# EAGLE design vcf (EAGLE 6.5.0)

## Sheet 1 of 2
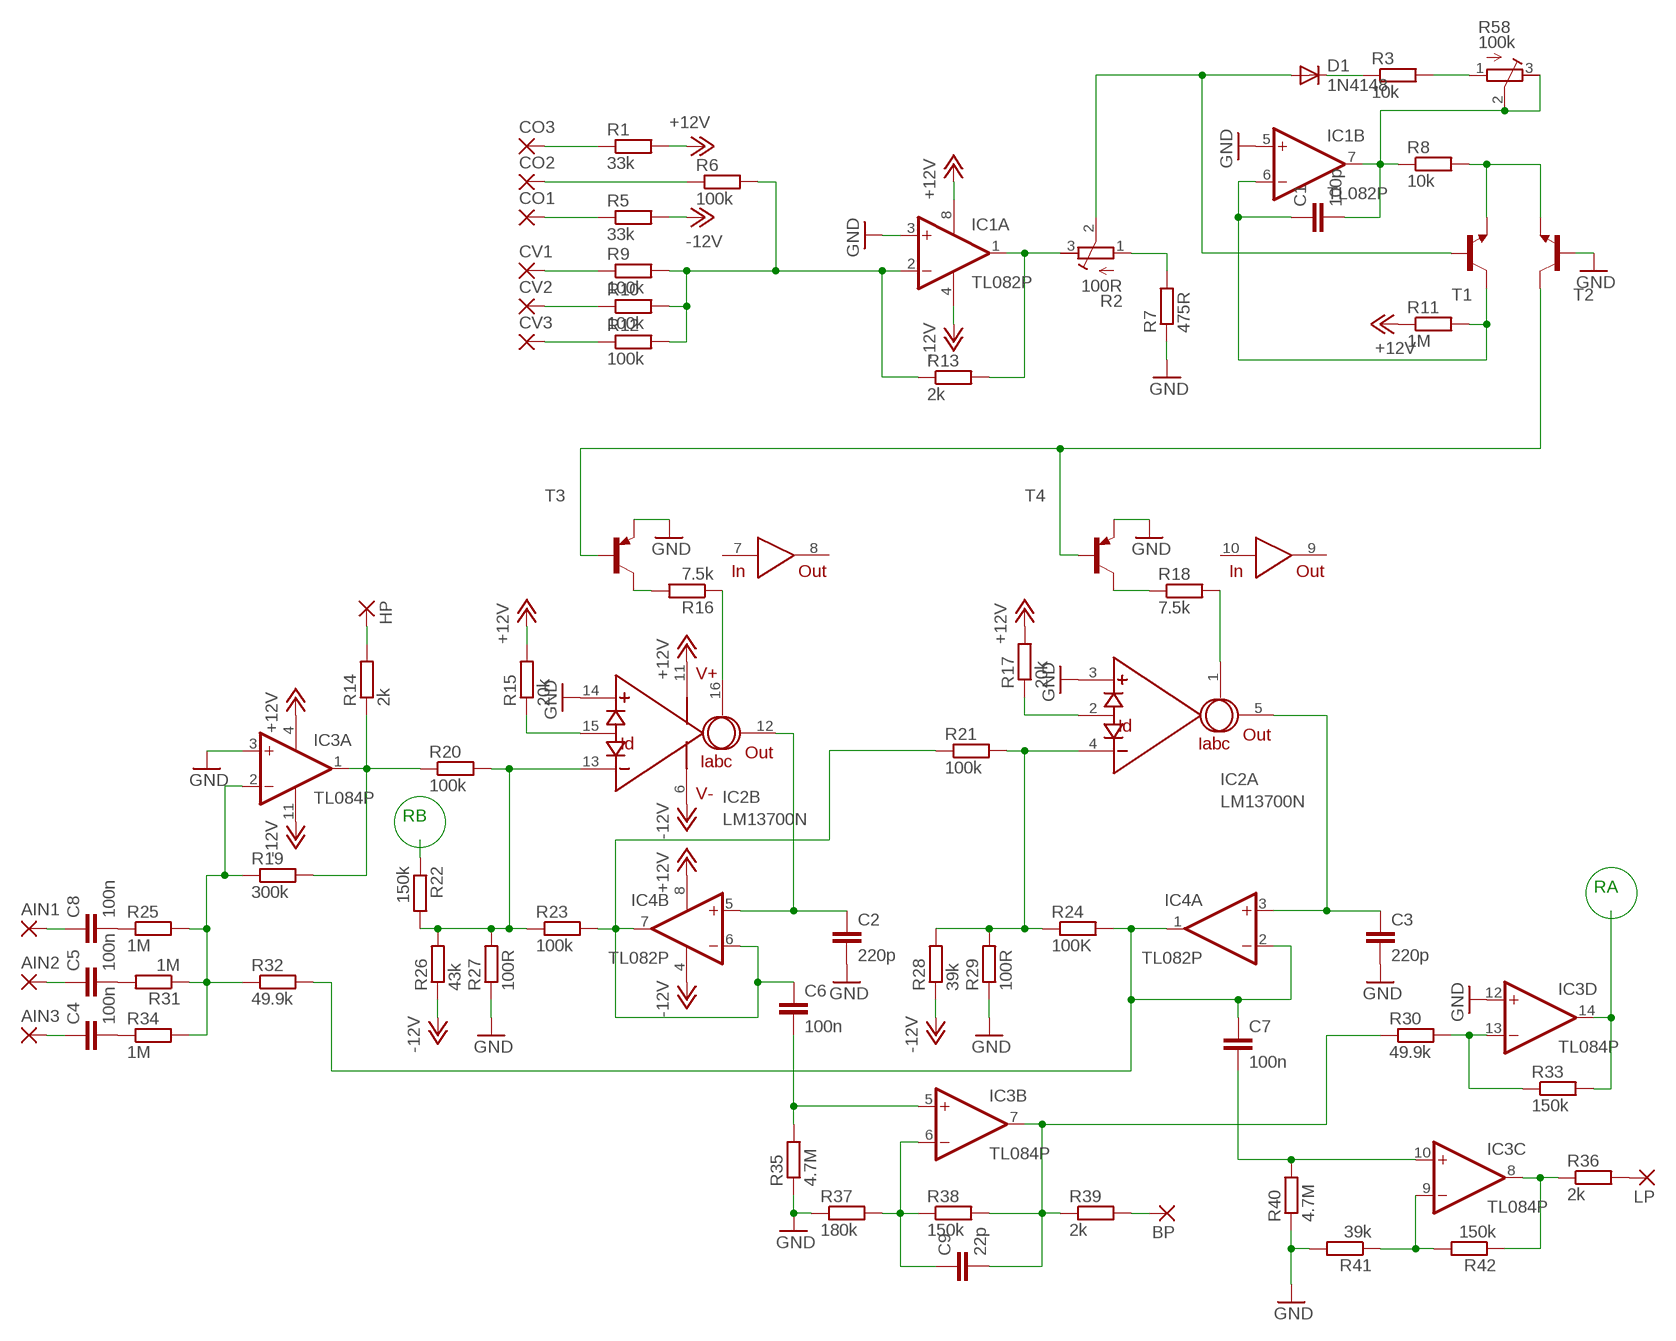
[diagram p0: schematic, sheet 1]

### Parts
AIN1  2,54/1,0  [2,54/1,0]
AIN2  2,54/1,0  [2,54/1,0]
AIN3  2,54/1,0  [2,54/1,0]
BP  2,54/1,0  [2,54/1,0]
C1  100p  C-EU050-035X075  [C050-035X075]
C2  220p  C-EU050-035X075  [C050-035X075]
C3  220p  C-EU050-035X075  [C050-035X075]
C4  100n  C-EU050-035X075  [C050-035X075]
C5  100n  C-EU050-035X075  [C050-035X075]
C6  100n  C-EU050-035X075  [C050-035X075]
C7  100n  C-EU050-035X075  [C050-035X075]
C8  100n  C-EU050-035X075  [C050-035X075]
C9  22p  C-EU050-035X075  [C050-035X075]
CO1  2,54/1,0  [2,54/1,0]
CO2  2,54/1,0  [2,54/1,0]
CO3  2,54/1,0  [2,54/1,0]
CV1  2,54/1,0  [2,54/1,0]
CV2  2,54/1,0  [2,54/1,0]
CV3  2,54/1,0  [2,54/1,0]
D1  1N4148  1N4148DO35-7  [DO35-7]
HP  2,54/1,0  [2,54/1,0]
IC1  TL082P  [DIL08]
IC2  LM13700N  [DIL16]
IC3  TL084P  [DIL14]
IC4  TL082P  [DIL08]
LP  2,54/1,0  [2,54/1,0]
R1  33k  R-EU_0309/10  [0309/10]
R2  100R  R-TRIMM64W  [RTRIM64W]
R3  10k  R-EU_0309/10  [0309/10]
R5  33k  R-EU_0309/10  [0309/10]
R6  100k  R-EU_0309/10  [0309/10]
R7  475R  R-EU_0309/10  [0309/10]
R8  10k  R-EU_0309/10  [0309/10]
R9  100k  R-EU_0309/10  [0309/10]
R10  100k  R-EU_0309/10  [0309/10]
R11  1M  R-EU_0309/10  [0309/10]
R12  100k  R-EU_0309/10  [0309/10]
R13  2k  R-EU_0309/10  [0309/10]
R14  2k  R-EU_0309/10  [0309/10]
R15  20k  R-EU_0309/10  [0309/10]
R16  7.5k  R-EU_0309/10  [0309/10]
R17  20k  R-EU_0309/10  [0309/10]
R18  7.5k  R-EU_0309/10  [0309/10]
R19  300k  R-EU_0309/10  [0309/10]
R20  100k  R-EU_0309/10  [0309/10]
R21  100k  R-EU_0309/10  [0309/10]
R22  150k  R-EU_0309/10  [0309/10]
R23  100k  R-EU_0309/10  [0309/10]
R24  100K  R-EU_0309/10  [0309/10]
R25  1M  R-EU_0309/10  [0309/10]
R26  43k  R-EU_0309/10  [0309/10]
R27  100R  R-EU_0309/10  [0309/10]
R28  39k  R-EU_0309/10  [0309/10]
R29  100R  R-EU_0309/10  [0309/10]
R30  49.9k  R-EU_0309/10  [0309/10]
R31  1M  R-EU_0309/10  [0309/10]
R32  49.9k  R-EU_0309/10  [0309/10]
R33  150k  R-EU_0309/10  [0309/10]
R34  1M  R-EU_0309/10  [0309/10]
R35  4.7M  R-EU_0309/10  [0309/10]
R36  2k  R-EU_0309/10  [0309/10]
R37  180k  R-EU_0309/10  [0309/10]
R38  150k  R-EU_0309/10  [0309/10]
R39  2k  R-EU_0309/10  [0309/10]
R40  4.7M  R-EU_0309/10  [0309/10]
R41  39k  R-EU_0309/10  [0309/10]
R42  150k  R-EU_0309/10  [0309/10]
R58  100k  R-TRIMM64W  [RTRIM64W]
T1  2N3904-NPN-TO92-EBC  [TO92-EBC]
T2  2N3904-NPN-TO92-EBC  [TO92-EBC]
T3  2N3906-PNP-TO92-EBC  [TO92-EBC]
T4  2N3906-PNP-TO92-EBC  [TO92-EBC]

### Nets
+12V: IC1.8(P:V+) IC2.11(V+) IC3.4(P:V+) IC4.8(P:V+) R1.2 R11.1 R15.2 R17.2 ; also sheet 2
-12V: IC1.4(P:V-) IC2.6(V-) IC3.11(P:V-) IC4.4(P:V-) R5.2 R26.1 R28.1 ; also sheet 2
GND: C2.2 C3.2 IC1.3(A:+IN) IC1.5(B:+IN) IC2.3(A:+IN) IC2.14(B:+IN) IC3.3(A:+IN) IC3.12(D:+IN) R7.1 R27.1 R29.1 R35.1 R37.1 R40.1 R41.2 T2.B T3.E T4.E ; also sheet 2
N$13: CO3.1(P) R1.1
N$14: CO2.1(P) R6.1
N$15: CO1.1(P) R5.1
N$16: CV1.1(P) R9.1
N$17: CV2.1(P) R10.1
N$18: CV3.1(P) R12.1
N$19: IC1.2(A:-IN) R6.2 R9.2 R10.2 R12.2 R13.1
N$20: IC1.1(A:OUT) R2.3(E) R13.2
N$21: R2.1(A) R7.2
N$22: C8.2 R25.1
N$23: R8.2 T1.E T2.E
N$24: C1.1 IC1.6(B:-IN) R11.2 T1.C
N$25: D1.C R3.1
N$26: R3.2 R58.1(A)
N$27: C1.2 IC1.7(B:OUT) R8.1 R58.2(S) R58.3(E)
N$28: D1.A R2.2(S) T1.B
N$29: T2.C T3.B T4.B
N$30: C6.2 IC3.5(B:+IN) R35.2
N$31: C5.2 R31.2
N$32: C4.2 R34.1
N$33: IC3.1(A:OUT) R14.1 R19.2 R20.1
N$34: HP.1(P) R14.2
N$35: IC3.2(A:-IN) R19.1 R25.2 R31.1 R32.1 R34.2
N$36: IC2.13(B:-IN) R20.2 R22.2 R23.1 R26.2 R27.2
N$37: IC2.15(B:ID) R15.1
N$38: IC2.2(A:ID) R17.1
N$39: IC2.16(B:IABC) R16.1
N$40: R16.2 T3.C
N$41: R18.1 T4.C
N$42: IC2.1(A:IABC) R18.2
N$43: IC2.4(A:-IN) R21.2 R24.1 R28.2 R29.2
N$44: C6.1 IC4.6(B:-IN) IC4.7(B:OUT) R21.1 R23.2
N$45: C2.1 IC2.12(B:OUT) IC4.5(B:+IN)
N$46: C3.1 IC2.5(A:OUT) IC4.3(A:+IN)
N$47: AIN1.1(P) C8.1
N$48: C9.1 IC3.6(B:-IN) R37.2 R38.1
N$50: C9.2 IC3.7(B:OUT) R30.1 R38.2 R39.1
N$51: BP.1(P) R39.2
N$52: IC3.13(D:-IN) R30.2 R33.1
N$53: AIN2.1(P) C5.1
N$54: C7.2 IC3.10(C:+IN) R40.2
N$55: IC3.9(C:-IN) R41.1 R42.2
N$56: IC3.8(C:OUT) R36.1 R42.1
N$57: LP.1(P) R36.2
N$58: AIN3.1(P) C4.1
N$59: C7.1 IC4.1(A:OUT) IC4.2(A:-IN) R24.2 R32.2
RA: IC3.14(D:OUT) R33.2 ; also sheet 2
RB: R22.1 ; also sheet 2
Unconnected: IC2.7(IN) IC2.8(OUT) IC2.9(OUT) IC2.10(IN)

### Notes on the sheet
- RB
- RA

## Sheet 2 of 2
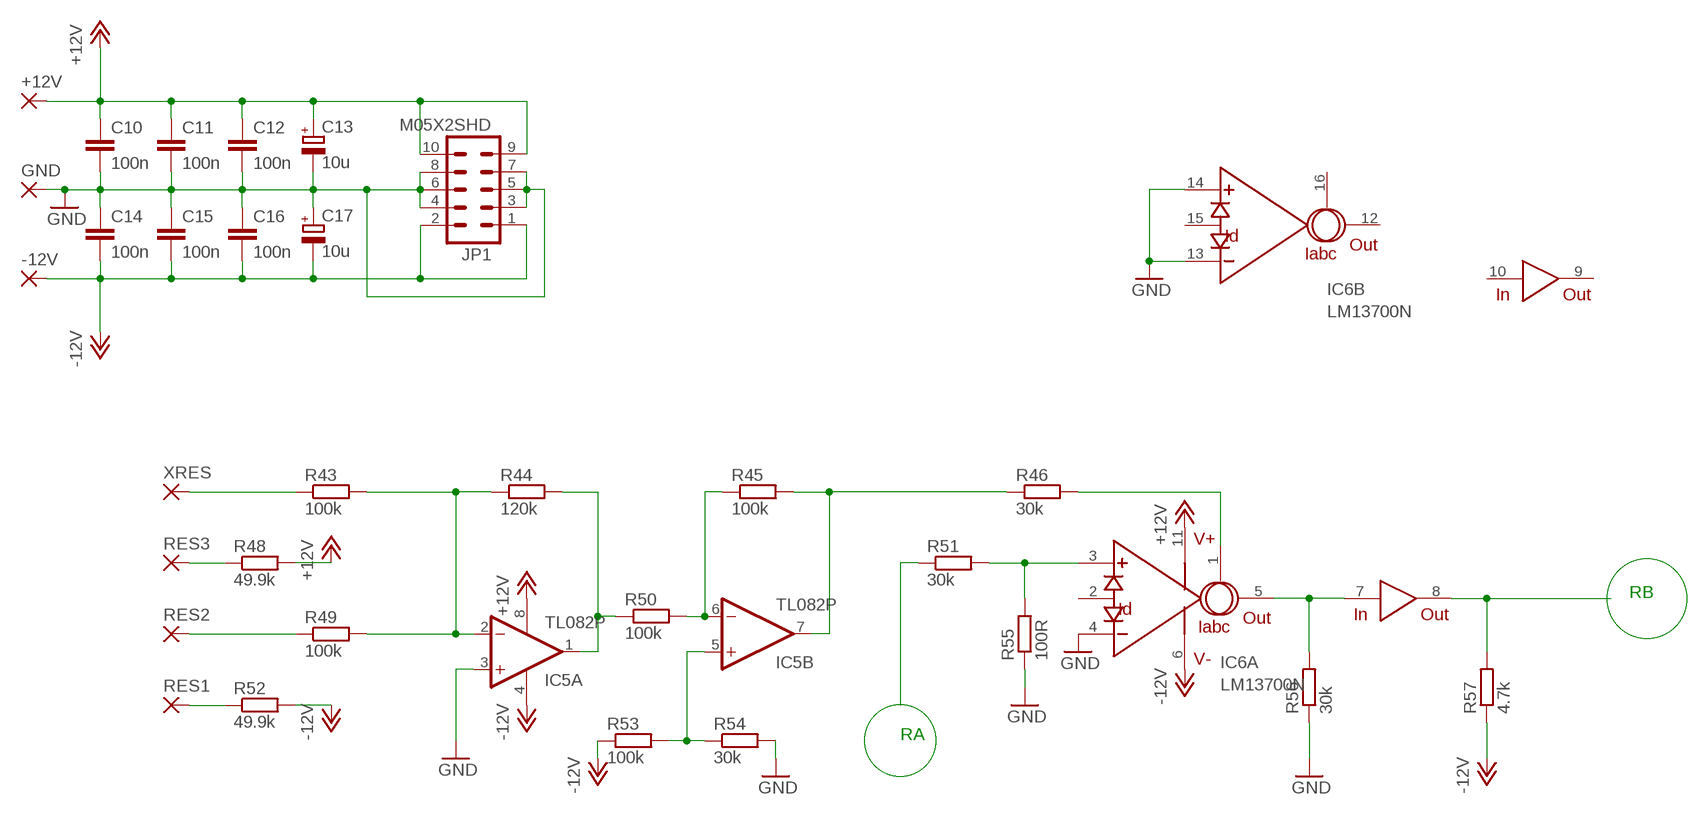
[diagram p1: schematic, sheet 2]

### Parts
+12V  2,54/1,0  [2,54/1,0]
-12V  2,54/1,0  [2,54/1,0]
C10  100n  C-EU050-035X075  [C050-035X075]
C11  100n  C-EU050-035X075  [C050-035X075]
C12  100n  C-EU050-035X075  [C050-035X075]
C13  10u  CPOL-EUE3.5-8  [E3,5-8]
C14  100n  C-EU050-035X075  [C050-035X075]
C15  100n  C-EU050-035X075  [C050-035X075]
C16  100n  C-EU050-035X075  [C050-035X075]
C17  10u  CPOL-EUE3.5-8  [E3,5-8]
GND  2,54/1,0  [2,54/1,0]
IC5  TL082P  [DIL08]
IC6  LM13700N  [DIL16]
JP1  M05X2SHD  [2X5-SHROUDED]
R43  100k  R-EU_0309/10  [0309/10]
R44  120k  R-EU_0309/10  [0309/10]
R45  100k  R-EU_0309/10  [0309/10]
R46  30k  R-EU_0309/10  [0309/10]
R48  49.9k  R-EU_0309/10  [0309/10]
R49  100k  R-EU_0309/10  [0309/10]
R50  100k  R-EU_0309/10  [0309/10]
R51  30k  R-EU_0309/10  [0309/10]
R52  49.9k  R-EU_0309/10  [0309/10]
R53  100k  R-EU_0309/10  [0309/10]
R54  30k  R-EU_0309/10  [0309/10]
R55  100R  R-EU_0309/10  [0309/10]
R56  30k  R-EU_0309/10  [0309/10]
R57  4.7k  R-EU_0309/10  [0309/10]
RES1  2,54/1,0  [2,54/1,0]
RES2  2,54/1,0  [2,54/1,0]
RES3  2,54/1,0  [2,54/1,0]
XRES  2,54/1,0  [2,54/1,0]

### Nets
+12V: +12V.1(P) C10.1 C11.1 C12.1 C13.+ IC5.8(P:V+) IC6.11(V+) JP1.9 JP1.10 R48.2 ; also sheet 1
-12V: -12V.1(P) C14.2 C15.2 C16.2 C17.- IC5.4(P:V-) IC6.6(V-) JP1.1 JP1.2 R52.2 R53.1 R57.1 ; also sheet 1
GND: C10.2 C11.2 C12.2 C13.- C14.1 C15.1 C16.1 C17.+ GND.1(P) IC5.3(A:+IN) IC6.4(A:-IN) IC6.13(B:-IN) IC6.14(B:+IN) JP1.3 JP1.4 JP1.5 JP1.6 JP1.7 JP1.8 R54.2 R55.1 R56.1 ; also sheet 1
N$1: R43.1 XRES.1(P)
N$2: R48.1 RES3.1(P)
N$3: R52.1 RES1.1(P)
N$4: R49.1 RES2.1(P)
N$5: IC5.2(A:-IN) R43.2 R44.1 R49.2
N$6: IC5.1(A:OUT) R44.2 R50.1
N$7: IC5.6(B:-IN) R45.1 R50.2
N$8: IC5.5(B:+IN) R53.2 R54.1
N$9: IC6.1(A:IABC) R46.2
N$10: IC5.7(B:OUT) R45.2 R46.1
N$11: IC6.3(A:+IN) R51.2 R55.2
N$12: IC6.5(A:OUT) IC6.7(IN) R56.2
RA: R51.1 ; also sheet 1
RB: IC6.8(OUT) R57.2 ; also sheet 1
Unconnected: IC6.2(A:ID) IC6.9(OUT) IC6.10(IN) IC6.12(B:OUT) IC6.15(B:ID) IC6.16(B:IABC)

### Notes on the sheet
- RB
- RA

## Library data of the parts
+12V -12V AIN1-AIN3 BP CO1-CO3 CV1-CV3 GND HP LP RES1-RES3 XRES = wirepad:2,54/1,0: THROUGH-HOLE PAD
C1-C12 C14-C16 = rcl:C-EU: CAPACITOR, European symbol
C13 C17 = rcl:CPOL-EU: POLARIZED CAPACITOR, European symbol
D1 = diode:1N4148: DIODE
IC1 IC4 IC5 = cavalier:TL082: OP AMP
IC2 IC6 = synthdiy:LM13700: National Dual OTA with buffers.
IC3 = cavalier:TL084: OP AMP
JP1 = SparkFun:M05X2: Header 5x2 Standard 10-pin dual row 0.1" header. Commonly used with AVR-ISP. Use with Spark Fun Electronics SKU: PRT-00778
R1 R3 R5-R46 R48-R57 = rcl:R-EU_: RESISTOR, European symbol
R2 R58 = rcl:R-TRIMM: Trimm resistor
T1 T2 = transistor-neu-to92:*-NPN-: NPN Transistror
T3 T4 = transistor-neu-to92:*-PNP-: PNP Transistror

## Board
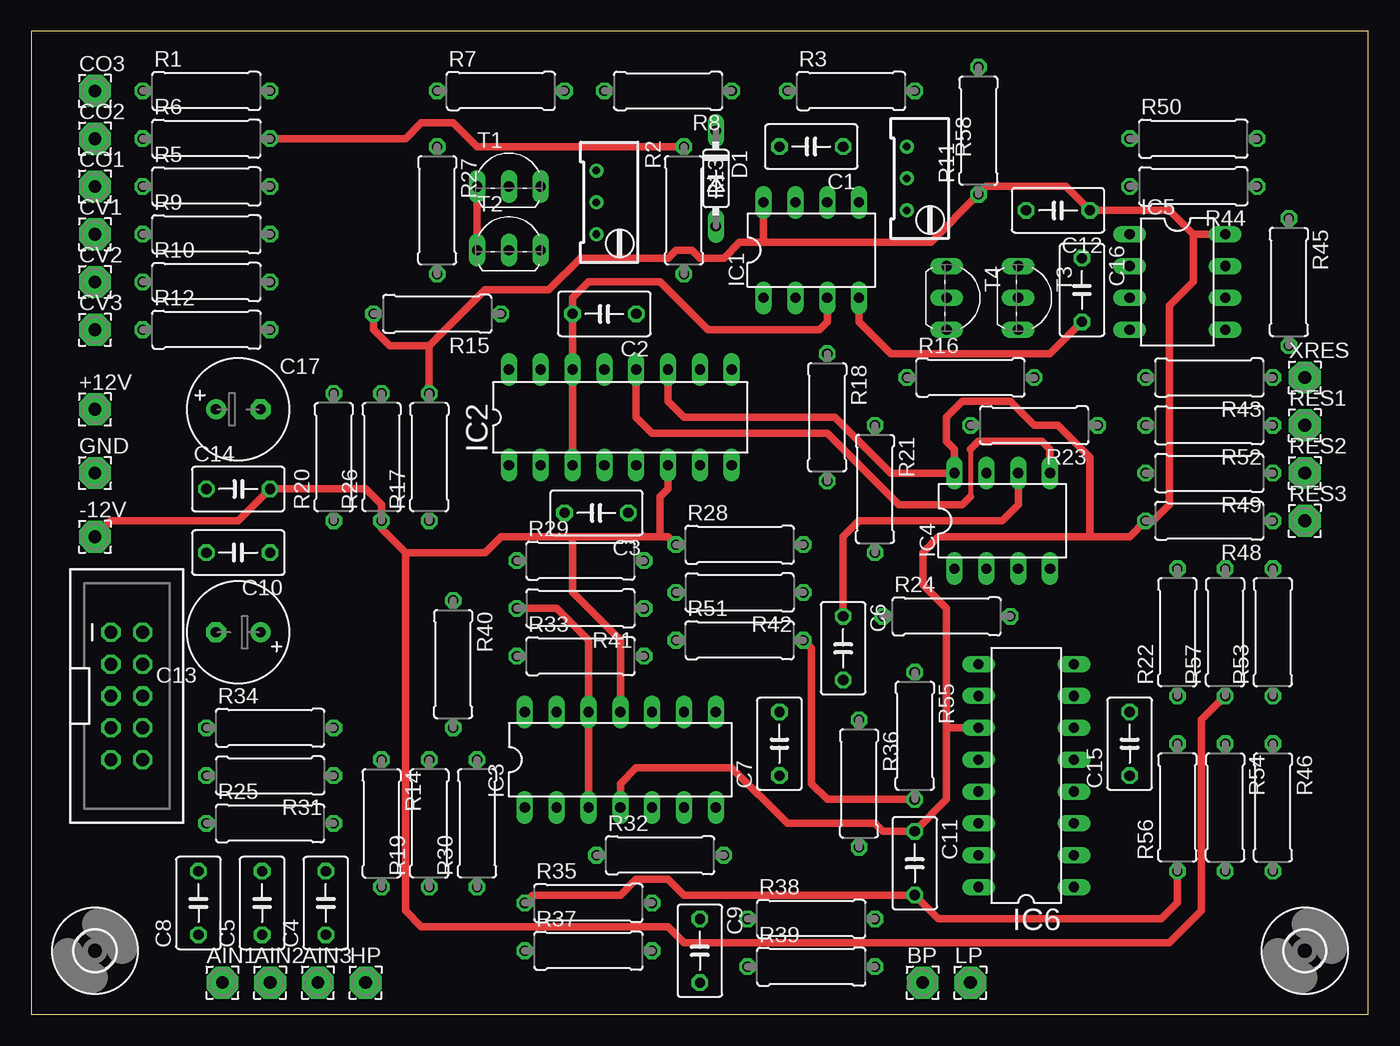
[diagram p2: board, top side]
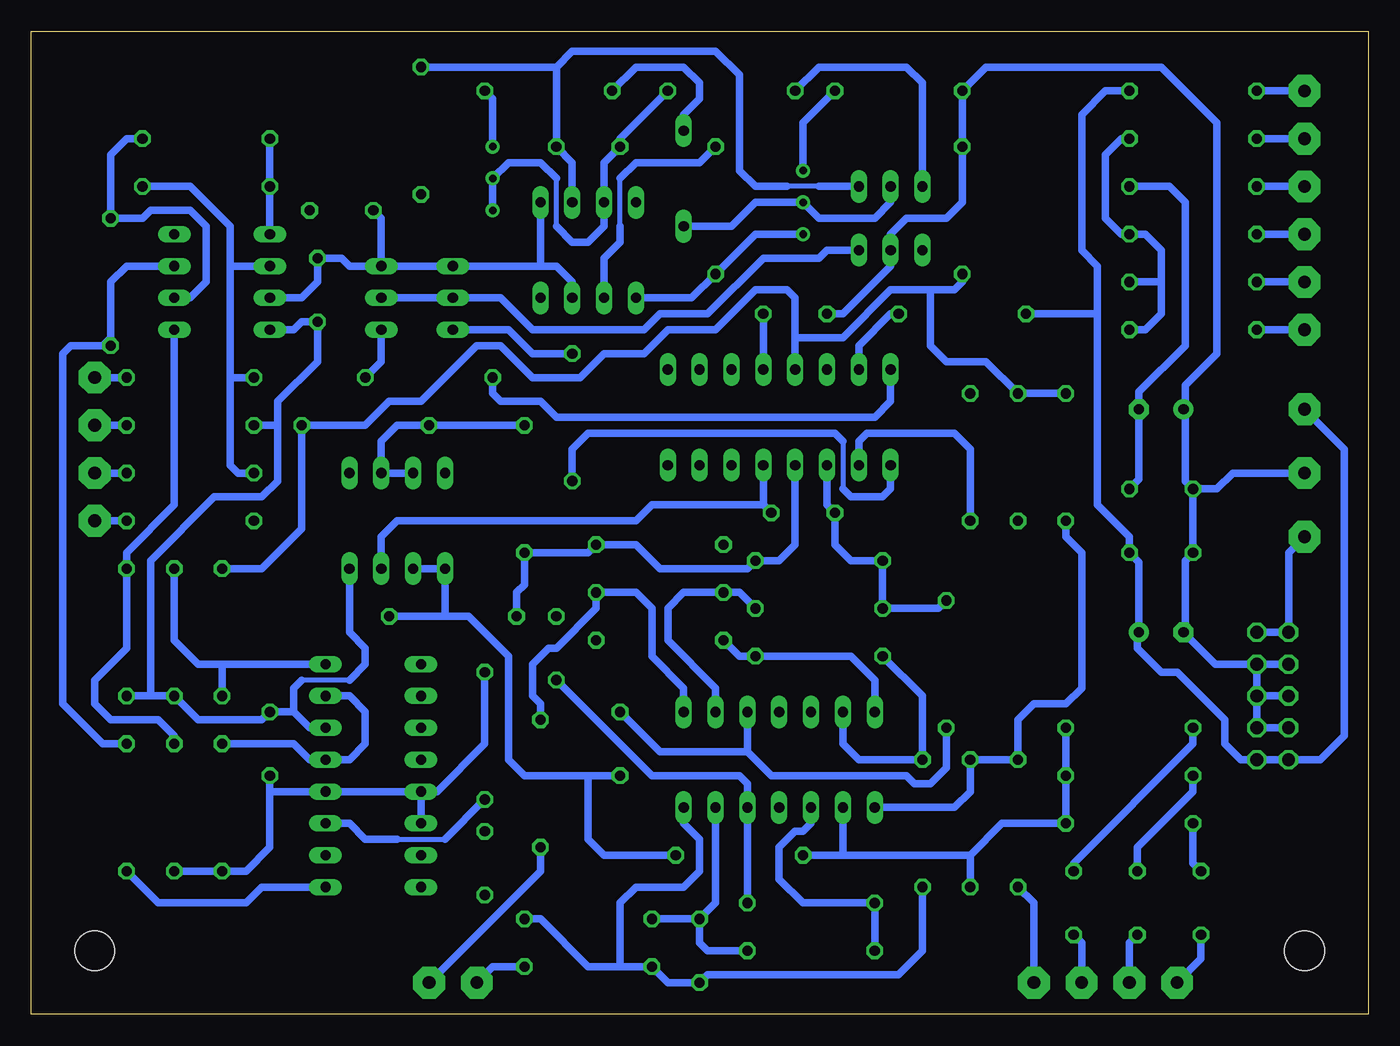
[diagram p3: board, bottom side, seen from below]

Size 106.66 x 78.41 mm. Coordinates in mm from the lower left corner, seen from the top.
Outline: 0,0 106.66,0 106.66,78.41 0,78.41 0,0
Copper layers (1*16): Top 0.035mm / dielectric 1.5mm / Bottom 0.035mm
Design rules "default": minimum track width 10mil, minimum drill 24mil, track to track 8mil, track to pad 8mil, pad to pad 8mil, via to via 8mil, smd to smd 8mil, copper to edge 40mil, drill to drill 8mil, minimum pad ring 10mil, minimum via ring 8mil, stop-mask expansion 4mil, vias tented up to drill 0mil, thermal gap 10mil

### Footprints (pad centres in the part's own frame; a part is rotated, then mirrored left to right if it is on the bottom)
2,54/1,0 = drill 1.016 pad 2.54 octagon: 1 0,0
C050-035X075 = drill 0.813 octagon: 1 -2.54,0; 2 2.54,0
E3,5-8 = drill 0.813 pad 1.6: + -1.778,0 | drill 0.813 pad 1.6 octagon: - 1.778,0
DO35-7 = drill 0.813 long: A 3.81,0; C -3.81,0
DIL08 = drill 0.813 pad 1.27 long: 1 -3.81,-3.81; 2 -1.27,-3.81; 3 1.27,-3.81; 4 3.81,-3.81; 5 3.81,3.81; 6 1.27,3.81; 7 -1.27,3.81; 8 -3.81,3.81
DIL16 = drill 0.813 long: 1 -8.89,-3.81; 2 -6.35,-3.81; 3 -3.81,-3.81; 4 -1.27,-3.81; 5 1.27,-3.81; 6 3.81,-3.81; 7 6.35,-3.81; 8 8.89,-3.81; 9 8.89,3.81; 10 6.35,3.81; 11 3.81,3.81; 12 1.27,3.81; 13 -1.27,3.81; 14 -3.81,3.81; 15 -6.35,3.81; 16 -8.89,3.81
DIL14 = drill 0.813 long: 1 -7.62,-3.81; 2 -5.08,-3.81; 3 -2.54,-3.81; 4 0,-3.81; 5 2.54,-3.81; 6 5.08,-3.81; 7 7.62,-3.81; 8 7.62,3.81; 9 5.08,3.81; 10 2.54,3.81; 11 0,3.81; 12 -2.54,3.81; 13 -5.08,3.81; 14 -7.62,3.81
2X5-SHROUDED = drill 1.016 octagon: 1 -1.27,5.08; 2 1.27,5.08; 3 -1.27,2.54; 4 1.27,2.54; 5 -1.27,0; 6 1.27,0; 7 -1.27,-2.54; 8 1.27,-2.54; 9 -1.27,-5.08; 10 1.27,-5.08
0309/10 = drill 0.813 octagon: 1 -5.08,0; 2 5.08,0
RTRIM64W = drill 0.61: 1 1.27,-2.54; 2 1.27,0; 3 1.27,2.54
TO92-EBC = drill 0.813 long: B 0,-1.27; C 2.54,-1.27; E -2.54,-1.27
3,2 = hole 3.2: 0,0

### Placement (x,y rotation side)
+12V  5.08,48.26 0 top
-12V  5.08,38.1 0 top
AIN1  15.24,2.54 0 top
AIN2  19.05,2.54 0 top
AIN3  22.86,2.54 0 top
BP  71.12,2.54 0 top
C1  62.23,69.22 180 top
C2  45.72,55.88 180 top
C3  45.09,40.01 180 top
C4  23.5,8.89 90 top
C5  18.41,8.89 90 top
C6  64.77,29.21 270 top
C7  59.69,21.59 90 top
C8  13.34,8.89 90 top
C9  53.34,5.08 270 top
C10  16.51,36.83 180 top
C11  70.48,12.06 270 top
C12  81.92,64.14 180 top
C13  16.51,30.48 180 top
C14  16.51,41.91 0 top
C15  87.63,21.59 90 top
C16  83.82,57.78 270 top
C17  16.51,48.26 0 top
CO1  5.08,66.04 0 top
CO2  5.08,69.85 0 top
CO3  5.08,73.66 0 top
CV1  5.08,62.23 0 top
CV2  5.08,58.42 0 top
CV3  5.08,54.61 0 top
D1  54.61,66.67 270 top
GND  5.08,43.18 0 top
HP  26.67,2.54 0 top
IC1  62.23,60.96 0 top
IC2  46.99,47.62 0 top
IC3  46.99,20.32 0 top
IC4  77.47,39.37 0 top
IC5  91.44,58.42 270 top
IC6  79.38,19.05 90 top
JP1  7.62,25.4 0 top
LP  74.93,2.54 0 top
R1  13.97,73.66 0 top
R2  46.35,64.77 180 top
R3  65.41,73.66 0 top
R5  13.97,66.04 0 top
R6  13.97,69.85 0 top
R7  37.47,73.66 0 top
R8  50.8,73.66 180 top
R9  13.97,62.23 0 top
R10  13.97,58.42 0 top
R11  75.56,70.48 90 top
R12  13.97,54.61 0 top
R13  52.07,64.14 270 top
R14  27.94,15.24 270 top
R15  32.38,55.88 180 top
R16  74.93,50.8 0 top
R17  31.75,44.45 90 top
R18  63.5,47.62 270 top
R19  31.75,15.24 90 top
R20  24.13,44.45 90 top
R21  67.31,41.91 270 top
R22  91.44,30.48 90 top
R23  80.01,46.99 180 top
R24  73.03,31.75 0 top
R25  19.05,15.24 0 top
R26  27.94,44.45 90 top
R27  32.38,64.14 270 top
R28  56.52,37.47 0 top
R29  43.81,36.2 0 top
R30  35.56,15.24 90 top
R31  19.05,19.05 180 top
R32  50.16,12.7 0 top
R33  43.81,28.57 0 top
R34  19.05,22.86 0 top
R35  44.45,8.89 0 top
R36  66.04,18.41 270 top
R37  44.45,5.08 0 top
R38  62.23,7.62 0 top
R39  62.23,3.81 0 top
R40  33.66,27.94 270 top
R41  43.81,32.38 180 top
R42  56.52,33.66 180 top
R43  93.98,50.8 180 top
R44  92.71,66.04 180 top
R45  100.33,58.42 270 top
R46  99.06,16.51 270 top
R48  93.98,39.37 180 top
R49  93.98,43.18 180 top
R50  92.71,69.85 0 top
R51  56.52,29.84 0 top
R52  93.98,46.99 180 top
R53  99.06,30.48 90 top
R54  95.25,16.51 270 top
R55  70.48,22.23 270 top
R56  91.44,16.51 90 top
R57  95.25,30.48 90 top
R58  71.12,66.67 180 top
RES1  101.6,46.99 0 top
RES2  101.6,43.18 0 top
RES3  101.6,39.37 0 top
T1  38.1,67.31 0 top
T2  38.1,62.23 0 top
T3  80.01,57.15 270 top
T4  74.3,57.15 270 top
U$1  [3,2]  5.08,5.08 0 top
U$2  [3,2]  101.6,5.08 0 top
XRES  101.6,50.8 0 top

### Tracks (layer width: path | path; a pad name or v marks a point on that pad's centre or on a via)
+12V
  Top 0.61: IC3.4 46.99,18.41 48.26,19.68 55.88,19.68 60.33,15.24 67.31,15.24 67.94,14.61 C11.1 73.03,17.14 73.03,22.86 | 73.03,22.86 73.03,32.38 71.12,34.29 71.12,36.83 72.39,38.1 84.45,38.1 | R15.2 27.3,54.61 28.57,53.34 31.75,53.34 | 92.71,62.23 90.81,64.14 C12.1 82.55,66.04 76.2,66.04 R11.1 71.75,61.59 58.42,61.59 | 92.71,62.23 IC5.8 | IC6.11 73.03,22.86 | 92.71,62.23 92.71,58.42 90.81,56.52 90.81,40.64 89.53,39.37 R48.2 87.63,38.1 84.45,38.1 | IC1.8 58.42,61.59 | IC2.11 50.8,48.9 52.07,47.62 64.14,47.62 68.58,43.18 IC4.8 73.66,45.09 73.03,45.72 73.03,47.62 74.3,48.9 78.11,48.9 80.01,46.99 81.92,46.99 84.45,44.45 84.45,38.1 | R17.2 31.75,53.34 | 58.42,61.59 56.52,61.59 55.24,60.33 53.34,60.33 52.7,60.96 51.44,60.96 50.8,60.33 43.81,60.33 41.27,57.78 36.2,57.78 31.75,53.34
  Bottom 0.61: +12V.1 1.91,45.09 1.91,22.23 3.81,20.32 JP1.9 JP1.10 10.16,20.32 11.43,21.59 11.43,23.5 15.24,27.3 16.51,27.3 18.41,29.21 18.41,30.35 C13.+ 18.29,36.07 C10.1 19.05,38.1 21.59,40.64 21.59,55.88 | 21.59,55.88 21.59,59.69 22.86,60.96 22.86,71.75 20.95,73.66 R1.2 | 21.59,55.88 R15.2
-12V
  Top 0.61: 29.84,36.83 36.2,36.83 37.47,38.1 43.18,38.1 | 43.18,38.1 50.16,38.1 | IC2.6 50.8,41.91 50.16,41.27 50.16,38.1 | IC3.11 46.99,29.84 43.18,33.66 43.18,38.1 | IC1.4 66.04,55.24 68.58,52.7 81.28,52.7 C16.2 | R57.1 93.34,23.5 93.34,8.26 90.81,5.71 52.07,5.71 50.8,6.99 31.11,6.99 29.84,8.26 29.84,36.83 | 50.16,38.1 50.8,38.1 R28.1 | 29.84,36.83 27.94,38.73 R26.1 27.94,40.64 26.67,41.91 C14.2 16.51,39.37 6.35,39.37 -12V.1
  Bottom 0.406: 81.28,26.67 85.09,26.67
  Bottom 0.61: JP1.2 JP1.1 6.35,36.83 -12V.1 | R53.1 97.16,25.4 | 97.16,25.4 R57.1 93.34,23.5 88.27,23.5 C15.2 85.72,24.13 | C14.2 18.29,42.67 C17.- 18.29,49.66 14.61,53.34 14.61,64.77 15.88,66.04 R5.2 | IC6.6 84.45,22.86 85.72,24.13 | R52.2 87,46.99 | 87,46.99 87,42.55 88.27,41.27 92.08,41.27 97.16,36.2 97.16,25.4 | IC4.4 81.28,30.48 80.01,29.21 80.01,27.94 81.28,26.67 | 85.09,26.67 85.72,26.04 85.72,24.13 | 87,46.99 87,48.9 83.82,52.07 C16.2 85.09,55.24 85.72,54.61 IC5.4
GND
  Top 0.61: IC3.3 IC3.12 44.45,29.84 41.91,32.38 R41.2 | R56.1 91.44,8.89 90.17,7.62 72.39,7.62 C11.2 52.07,9.53 50.8,10.79 48.26,10.79 46.99,9.53 40.01,9.53 R35.1 | IC2.3 IC2.14 C2.2 43.18,57.15 44.45,58.42 50.16,58.42 53.98,54.61 62.87,54.61 63.5,55.24 IC1.3
  Bottom 0.61: JP1.7 JP1.8 JP1.6 | JP1.5 JP1.6 | JP1.3 JP1.4 | JP1.6 JP1.4 | R37.1 R35.1 45.09,8.89 46.99,10.79 46.99,13.34 45.72,14.61 45.09,14.61 44.45,15.24 IC3.3 | R54.2 R56.1 89.53,11.43 87.63,13.34 87.63,17.78 | IC6.13 IC6.4 87.63,17.78 | IC6.13 IC6.14 | IC6.13 74.3,17.78 70.48,21.59 R55.1 | T3.E T4.E 66.04,59.69 | 66.04,59.69 64.77,59.69 63.5,58.42 IC1.3 | IC1.5 66.04,59.69 | GND.1 10.79,43.18 12.06,41.91 C14.1 | C14.1 C10.2 14.61,36.2 14.61,30.61 C13.- 12.19,27.94 JP1.4 | C14.1 14.61,42.55 14.61,48.13 C17.+ 14.61,48.26 14.61,50.16 12.06,52.7 12.06,71.12 16.51,75.56 30.48,75.56 R7.1 R27.1 32.38,64.77 33.66,63.5 36.83,63.5 38.1,62.23 T2.B 38.1,59.69 41.91,55.88 C2.2 | R40.1 34.29,32.38 R41.2 R29.1 41.27,36.2 42.55,37.47 C3.2 43.18,40.64 IC2.3 | C12.2 78.74,63.5 T3.E | IC5.3 85.09,57.15 83.82,58.42 C16.1 81.92,60.33 81.28,59.69 T3.E | 87.63,17.78 C15.1
N$1
  Bottom 0.61: XRES.1 R43.1
N$2
  Bottom 0.61: RES3.1 R48.1
N$3
  Bottom 0.61: RES1.1 R52.1
N$4
  Bottom 0.61: RES2.1 R49.1
N$5
  Bottom 0.61: R44.1 93.98,66.04 90.81,62.87 90.81,59.69 | IC5.2 90.81,59.69 | 90.81,59.69 90.81,50.8 | 90.81,50.8 R43.2 | R49.2 90.17,43.18 90.81,43.81 90.81,50.8
N$6
  Bottom 0.61: IC5.1 R44.2 R50.1
N$7
  Bottom 0.61: IC5.6 93.98,57.15 92.71,58.42 92.71,62.87 93.98,64.14 97.16,64.14 97.79,63.5 R45.1 100.33,68.58 99.06,69.85 R50.2
N$8
  Bottom 0.61: R54.1 95.25,22.23 96.52,23.5 100.33,23.5 101.6,24.77 101.6,26.67 99.06,29.21 R53.2 99.06,36.83 95.25,40.64 IC5.5
N$9
  Bottom 0.61: IC6.1 88.27,10.16 89.53,8.89 96.52,8.89 R46.2
N$10
  Bottom 0.61: R46.1 100.97,21.59 104.14,24.77 104.14,52.7 103.5,53.34 100.97,53.34 | 100.97,53.34 R45.2 | IC5.7 99.06,59.69 100.33,58.42 100.33,53.98 100.97,53.34
N$11
  Top 0.61: R55.2 63.5,17.14 62.23,18.41 62.23,29.21 R51.2
  Bottom 0.406: 77.47,13.97 73.66,13.97
  Bottom 0.61: IC6.3 81.28,15.24 80.01,13.97 77.47,13.97 | 73.66,13.97 R55.2
N$12
  Bottom 0.61: R56.2 85.72,21.59 84.45,20.32 IC6.5 81.28,20.32 80.01,21.59 80.01,24.13 81.28,25.4 IC6.7
N$13
  Bottom 0.61: CO3.1 R1.1
N$14
  Bottom 0.61: CO2.1 R6.1
N$15
  Bottom 0.61: CO1.1 R5.1
N$16
  Bottom 0.61: CV1.1 R9.1
N$17
  Bottom 0.61: CV2.1 R10.1
N$18
  Bottom 0.61: CV3.1 R12.1
N$19
  Top 0.61: R6.2 29.84,69.85 31.11,71.12 33.66,71.12 35.56,69.22 R13.1
  Bottom 0.406: 59.69,62.87 59.69,66.67
  Bottom 0.61: IC1.2 60.96,60.33 59.69,61.59 59.69,62.87 | 59.69,66.67 58.42,67.94 53.34,67.94 R13.1 | 16.51,58.42 16.51,55.88 17.78,54.61 R12.2 | R10.2 16.51,58.42 | 16.51,58.42 16.51,60.96 17.78,62.23 R9.2 19.68,62.23 20.95,63.5 20.95,68.58 19.68,69.85 R6.2
N$20
  Bottom 0.61: R2.3 48.9,62.23 R13.2 53.98,57.15 IC1.1
N$21
  Bottom 0.61: R2.1 45.09,71.12 R7.2
N$22
  Bottom 0.61: R25.1 13.97,12.06 C8.2
N$23
  Top 0.61: T2.E T1.E
  Bottom 0.61: T1.E 35.56,74.3 36.83,75.56 43.81,75.56 R8.2
N$24
  Bottom 0.406: 43.81,66.04 46.35,66.04
  Bottom 0.61: 64.77,75.56 C1.1 63.5,67.94 IC1.6 | 64.77,75.56 63.5,76.83 52.07,76.83 50.16,74.93 50.16,67.31 48.9,66.04 46.35,66.04 | T1.C 43.81,66.04 | R11.2 64.77,75.56
N$25
  Bottom 0.61: D1.C 54.61,71.75 53.34,73.03 53.34,74.3 54.61,75.56 58.42,75.56 R3.1
N$26
  Bottom 0.61: R58.1 69.85,73.03 R3.2
N$27
  Bottom 0.406: 64.77,62.87 64.77,66.67
  Bottom 0.61: R58.3 R58.2 68.58,67.94 66.04,67.94 64.77,66.67 | R8.1 59.69,69.85 C1.2 60.96,67.94 IC1.7 60.96,62.87 62.23,61.59 63.5,61.59 64.77,62.87
N$28
  Bottom 0.61: T1.B 38.1,64.77 39.37,63.5 43.81,63.5 R2.2 48.9,64.77 50.8,62.87 D1.A
N$29
  Bottom 0.61: T2.C 43.18,60.96 43.81,60.33 48.26,60.33 52.7,55.88 56.52,55.88 57.78,54.61 66.67,54.61 69.22,57.15 T4.B T3.B
N$30
  Bottom 0.61: R35.2 IC3.5 49.53,18.41 50.16,19.05 57.15,19.05 C6.2
N$31
  Bottom 0.61: R31.2 13.97,17.78 18.41,13.34 C5.2
N$32
  Bottom 0.61: C4.2 23.5,12.06 13.97,21.59 R34.1
N$33
  Bottom 0.61: IC3.1 33.02,16.51 31.75,17.78 R19.2 R14.1 27.94,23.5 26.67,24.77 24.13,24.77 22.86,26.04 22.86,36.83 24.13,38.1 R20.1
N$34
  Bottom 0.61: HP.1 26.67,8.89 R14.2
N$35
  Bottom 0.61: R34.2 R31.1 R25.2 29.21,15.24 31.75,12.7 | R19.1 31.75,12.7 | 31.75,12.7 41.91,12.7 | 41.91,12.7 R32.1 | IC3.2 41.91,12.7
N$36
  Bottom 0.61: R20.2 R26.2 30.48,52.07 33.66,52.07 34.92,53.34 34.92,57.78 | 34.92,57.78 38.1,57.78 41.91,53.98 45.72,53.98 | 45.72,53.98 IC2.13 | 45.72,53.98 45.72,57.15 46.35,57.78 48.9,57.78 52.07,54.61 55.88,54.61 57.78,52.7 60.96,52.7 62.87,50.8 66.67,50.8 69.22,53.34 71.12,53.34 75.56,48.9 78.11,48.9 80.01,46.99 R23.1 85.09,38.73 88.27,35.56 R22.2 | R27.2 32.38,58.42 33.02,57.78 34.92,57.78
N$37
  Bottom 0.61: R15.1 38.1,55.88 40.64,53.34 IC2.15
N$38
  Bottom 0.61: R17.1 31.75,45.09 33.02,46.35 40.01,46.35 40.64,45.72 IC2.2
N$39
  Bottom 0.61: IC2.16 38.1,48.9 39.37,47.62 64.77,47.62 66.04,48.9 69.22,48.9 69.85,49.53 R16.1
N$40
  Bottom 0.61: T3.C 78.74,52.07 R16.2
N$41
  Bottom 0.61: R18.1 66.67,52.7 68.58,54.61 T4.C
N$42
  Bottom 0.406: 41.91,45.72 41.91,41.91
  Bottom 0.61: 41.91,45.72 42.55,46.35 62.23,46.35 63.5,45.09 R18.2 | 41.91,41.91 41.27,41.27 38.73,41.27 38.1,41.91 IC2.1
N$43
  Bottom 0.61: R24.1 67.94,33.66 67.31,34.29 R21.2 62.23,36.83 R28.2 58.42,37.47 56.52,35.56 49.53,35.56 R29.2 46.99,36.2 45.72,37.47 IC2.4
N$44
  Top 0.61: C6.1 64.77,38.1 66.04,39.37 77.47,39.37 78.74,40.64 IC4.6
  Bottom 0.61: IC4.7 IC4.6 78.74,45.72 77.47,46.99 R23.2 R21.1
N$45
  Top 0.406: 74.93,45.09 74.93,41.27
  Top 0.61: IC2.12 48.26,47.62 49.53,46.35 63.5,46.35 69.22,40.64 74.3,40.64 74.93,41.27 | IC4.5 81.28,45.09 80.64,45.72 75.56,45.72 74.93,45.09
  Bottom 0.61: C2.1 IC2.12
N$46
  Bottom 0.61: IC2.5 48.26,40.64 | 48.26,40.64 C3.1 | 48.26,40.64 57.15,40.64 58.42,39.37 77.47,39.37 78.74,38.1 IC4.3
N$47
  Bottom 0.61: C8.1 13.34,4.45 AIN1.1
N$48
  Bottom 0.61: IC3.6 52.07,8.89 C9.1 | R38.1 C9.1 | R37.2 52.7,5.08 53.34,5.71 C9.1
N$50
  Bottom 0.61: R30.1 35.56,5.08 37.47,3.17 52.7,3.17 C9.2 55.88,2.54 R39.1 59.69,3.81 | IC3.7 54.61,15.24 53.34,13.97 53.34,11.43 54.61,10.16 58.42,10.16 59.69,8.89 59.69,3.81 | R38.2 66.04,7.62 62.23,3.81 59.69,3.81
N$51
  Bottom 0.61: R39.2 69.85,3.81 BP.1
N$52
  Bottom 0.61: IC3.13 41.91,21.59 40.64,20.32 R30.2 35.56,25.4 R33.1
N$53
  Bottom 0.61: C5.1 19.05,5.71 AIN2.1
N$54
  Bottom 0.61: R40.2 33.66,19.68 34.92,18.41 36.2,18.41 36.83,19.05 47.62,19.05 49.53,20.95 | 49.53,20.95 IC3.10 | C7.2 56.52,20.95 49.53,20.95
N$55
  Bottom 0.61: IC3.9 52.07,26.04 55.88,29.84 55.88,32.38 54.61,33.66 R42.2 50.16,33.66 R41.1
N$56
  Bottom 0.61: IC3.8 54.61,26.04 57.15,28.57 57.15,32.38 58.42,33.66 R42.1 61.59,32.38 64.77,29.21 65.41,29.21 66.67,27.94 66.67,25.4 66.04,24.77 R36.1
N$57
  Bottom 0.61: R36.2 66.04,11.43 LP.1
N$58
  Bottom 0.61: C4.1 22.86,5.71 AIN3.1
N$59
  Bottom 0.61: R32.2 60.96,12.7 62.23,13.97 62.23,19.05 | C7.1 62.23,19.05 | 62.23,19.05 67.31,19.05 68.58,20.32 68.58,28.57 71.75,31.75 73.66,31.75 | 73.66,31.75 IC4.1 IC4.2 | R24.2 73.66,31.75
RA
  Bottom 0.61: IC3.14 39.37,26.67 41.27,28.57 R33.2 50.16,28.57 R51.1
RB
  Bottom 0.61: IC6.8 91.44,27.94 | 91.44,27.94 93.34,27.94 95.25,29.84 R57.2 | R22.1 91.44,27.94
